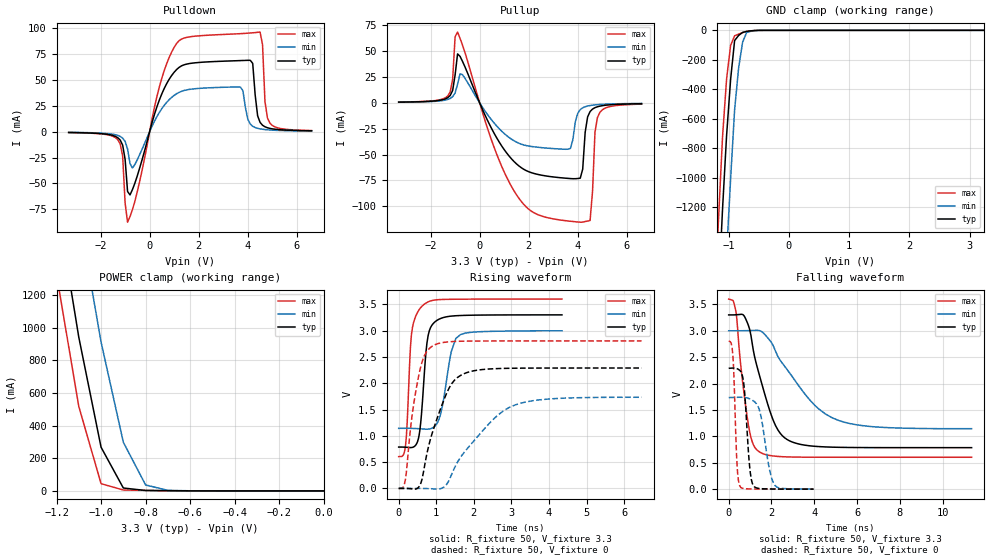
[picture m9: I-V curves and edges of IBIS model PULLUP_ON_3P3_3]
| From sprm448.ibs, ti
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|BUFFER OPERATING IN NORMAL MODE
|   Model Cell PULLUP_ON_3P3
|PULLUP_ON_3P3
[Model]   PULLUP_ON_3P3_3
Model_type   I/O
Polarity   Non-Inverting
Enable   Active-Low
Vinl =  0.8v
Vinh =  2v
Cref =  15.0000pF
Rref =  100.0000M
Vref =  0V
Vmeas =  1.65
C_comp   2.5107p   2.136p   3.1702p
[Model Spec]
Vinl   0.8v   0.8v   0.8v
Vinh   2v   2v   2v
[Temperature Range]   25   125   -40
[Voltage Range]   3.3   3   3.6
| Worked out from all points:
|   slope of the pulldown table from 0 to 0.495 V, typ, clamps not added: 13.6 ohm
|   slope of the pullup table from 0 to 0.495 V, typ, clamps not added: 19.6 ohm
|   GND clamp passes 1 mA (typ) near -0.54 V on its own axis
|   POWER clamp passes 1 mA (typ) near -0.67 V on its own axis
|   rising waveform, R_fixture 50, V_fixture 3.3: 20-80 % time 168ps typ, 264ps min, 133ps max; typ from 0.787 V to 3.3 V
|   rising waveform, R_fixture 50, V_fixture 0: 20-80 % time 594ps typ, 1.17ns min, 327ps max; typ from 0.001 V to 2.29 V
|   falling waveform, R_fixture 50, V_fixture 3.3: 20-80 % time 1.01ns typ, 2.05ns min, 503ps max; typ from 3.3 V to 0.787 V
|   falling waveform, R_fixture 50, V_fixture 0: 20-80 % time 228ps typ, 419ps min, 144ps max; typ from 2.29 V to 0.002 V
[POWER_clamp]
|   voltage   I(typ)   I(min)   I(max)
-3.3V     22.13A     22.81A     21.76A
-1.2V     1.777A     2.558A     1.326A
-1.167V   1.499A     2.271A     1.056A
-1.133V   1.22A      1.985A     786.8mA
-1.1V     941.2mA    1.698A     517.2mA
-1.067V   716.7mA    1.436A     359.6mA
-1.033V   492.2mA    1.174A     202mA
-1V       267.6mA    912.2mA    44.44mA
-900mV    17.9mA     298.1mA    5.577mA
-800mV    2.671mA    36.54mA    3.208mA
-700mV    1.259mA    3.427mA    1.602mA
-11.55fV  42.09pA    6.147nA    532.9fA
[Pulldown]
|   voltage   I(typ)   I(min)   I(max)
-3.3V     -841.7uA   -670.2uA   -911.7uA
-1.3V     -5.852mA   -3.631mA   -7.719mA
-1.1V     -12.99mA   -6.251mA   -23.52mA
-900mV    -57.7mA    -16.72mA   -87.34mA
-700mV    -55.82mA   -35.09mA   -75.1mA
1.1V      59.92mA    36.57mA    85.06mA
3.7V      68.51mA    42.92mA    94.48mA
4.1V      68.79mA    7.363mA    95.13mA
4.5V      8.911mA    2.645mA    95.99mA
4.7V      4.671mA    1.979mA    28.89mA
4.9V      3.124mA    1.577mA    8.243mA
6.6V      798.5uA    571.1uA    1.034mA
[Pullup]
|   voltage   I(typ)   I(min)   I(max)
-3.3V     669.2uA    562.7uA    746.5uA
-1.3V     4.957mA    3.264mA    6.677mA
-1.1V     12mA       5.961mA    22.79mA
-1V       26.99mA    9.54mA     64.01mA
-900mV    47.32mA    18.06mA    68.43mA
1.5V      -59.02mA   -37.98mA   -88.89mA
3.7V      -73.26mA   -44.09mA   -114.6mA
4.1V      -72.87mA   -6.563mA   -115.5mA
4.5V      -8.455mA   -2.591mA   -113.8mA
4.7V      -4.668mA   -1.97mA    -28.57mA
4.9V      -3.189mA   -1.585mA   -9.198mA
6.6V      -843.6uA   -589.3uA   -1.225mA
[GND_clamp]
|   voltage   I(typ)   I(min)   I(max)
-3.3V     -22.45A    -23.24A    -22.02A
-1.233V   -2.371A    -3.249A    -1.858A
-1.167V   -1.783A    -2.654A    -1.277A
-1.1V     -1.21A     -2.069A    -720.1mA
-1.033V   -714.5mA   -1.52A     -330.8mA
-966.7mV  -334.3mA   -1.01A     -103.1mA
-900mV    -69.19mA   -538.9mA   -36.95mA
-833.3mV  -34.75mA   -254.1mA   -25.5mA
-766.7mV  -14.11mA   -79.26mA   -15.67mA
-700mV    -7.271mA   -14.49mA   -7.449mA
-433.3mV  -189.2uA   -334.1uA   -218.7uA
3.233V    -5.66uA    14.7uA     -45.87uA
[Ramp]
| variable   typ   min   max
dV/dt_f   1.514821/1.012936n   1.118985/2.053563n   1.806692/0.503417n
dV/dt_r   1.381646/0.5943032n   1.0486/1.177325n   1.69059/0.3263678n
R_load = 50
[Rising Waveform]
R_fixture = 50
V_fixture = 3.3
V_fixture_min = 3
V_fixture_max = 3.6
|   time   V(typ)   V(min)   V(max)
0s        787.2mV    1.143V     605.4mV
184ps     784.2mV    1.144V     829.4mV
368ps     781.8mV    1.142V     3.063V
528ps     956.1mV    1.136V     3.379V
632ps     1.648V     1.132V     3.471V
784ps     2.908V     1.128V     3.546V
1.04ns    3.204V     1.262V     3.588V
1.4ns     3.276V     2.602V     3.596V
1.648ns   3.287V     2.925V     3.597V
4.344ns   3.299V     2.997V     3.6V
[Rising Waveform]
R_fixture = 50
V_fixture = 0
V_fixture_min = 0
V_fixture_max = 0
|   time   V(typ)   V(min)   V(max)
0s        997.8uV    886.7uV    1.259mV
184ps     1.513mV    1.022mV    189.7mV
344ps     -6.436mV   1.178mV    1.313V
552ps     45.45mV    1.318mV    2.206V
912ps     1.096V     -6.903mV   2.712V
1.416ns   1.997V     279.1mV    2.792V
1.888ns   2.219V     810.8mV    2.801V
2.624ns   2.279V     1.384V     2.803V
3.264ns   2.287V     1.624V     2.804V
6.464ns   2.29V      1.733V     2.804V
[Falling Waveform]
R_fixture = 50
V_fixture = 3.3
V_fixture_min = 3
V_fixture_max = 3.6
|   time   V(typ)   V(min)   V(max)
0s        3.3V       3V         3.6V
352ps     3.303V     3V         3.329V
768ps     3.248V     3.002V     1.653V
1.04ns    2.915V     3.004V     981.2mV
1.448ns   2.142V     3.002V     704.2mV
2.192ns   1.203V     2.61V      624.8mV
3.048ns   882.9mV    2.087V     609.3mV
4.216ns   807.4mV    1.518V     605.9mV
5.408ns   791.9mV    1.268V     605.5mV
11.35ns   787.3mV    1.146V     605.4mV
[Falling Waveform]
R_fixture = 50
V_fixture = 0
V_fixture_min = 0
V_fixture_max = 0
|   time   V(typ)   V(min)   V(max)
0s        2.29V      1.736V     2.804V
192ps     2.294V     1.737V     2.548V
400ps     2.28V      1.74V      402.3mV
544ps     2.239V     1.741V     46.06mV
720ps     1.947V     1.738V     12.44mV
960ps     511.3mV    1.715V     6.587mV
1.152ns   69.78mV    1.674V     4.895mV
1.48ns    12.21mV    1.434V     3.467mV
2.168ns   4.113mV    69.76mV    2.083mV
3.968ns   1.682mV    3.91mV     1.381mV
